| TEXAS INSTRUMENTS INCORPORATED
| Standard Linear and Logic Group
| IBIS Model of PCA9548A
| 8-CHANNEL I2C SWITCH WITH RESET
| This file contains package information for the following:
|  QFN 24-pin (RGE) package as [Component] PCA9548A_RGE
|  TSSOP 24-pin (PW) package as [Component] PCA9548A_PW
|  SOIC 24-pin (DW) package as [Component] PCA9548A_DW
|  TVSOP 24-pin (DGV) package as [Component] PCA9548A_DGV
|  SSOP 24-pin (DB) package as [Component] PCA9548A_DB
| This device can be powered at the following Vccs:
|  5 volt Vcc
|  3.3 volt Vcc
|  2.5 volt Vcc
| This file provides unique models under the [Model Selector] for each Vcc.
| For operation at a specific Vcc, select the appropriate model after each
| [Model Selector] keyword.
[IBIS Ver]   3.2
[Comment char]  |_char
[File Name]   pca9548a.ibs
[File Rev]   1.1 | a_die
[Date]   January 23, 2008
[Source]   Data created from TI-SPICE simulations at TI-SLL.
[Notes]   The following is an IBIS list for the PCA9548A.
   Please contact sllibis@ti.com with questions and
   comments concerning SLL IBIS models.
   - FILE REV HISTORY
   - 1.1 Release IBIS file on 1/23/08
   - Power clamp data has been deleted in all models except
   SDA terminator models as there is no power-clamp diode.
   - Non-monotonic data due to FET characteristics.
[Disclaimer] Property of Texas Instruments Incorporated.  Unauthorized
   reproduction and/or distribution is strictly prohibited.
   This product is protected under copyright law.
   Created  2007, (C) Copyright  2008, Texas Instruments
   Incorporated, All Rights Reserved
   UNLESS THERE IS A SIGNED, WRITTEN AGREEMENT TO THE
   CONTRARY, TEXAS INSTRUMENTS (TI) IS PROVIDING THE IBIS
   MODELS  AND WITHOUT ANY WARRANTY, EXPRESSED OR
   IMPLIED.  TI assumes no liability for:
   1) the accuracy of the IBIS models provided to your
   company;
   2) the proper functioning of these IBIS Models in your
   design or for any resulting applications; or
   3) infringement of patents, copyrights or intellectual
   property rights resulting from your use of these IBIS
   models.
   TI provides IBIS Models as a service to our customers.
   You and your company shall not distribute, sell or give
   these models to anyone else without prior written
   permission from TI.
   TI reserves the right to make changes to our products or
   to discontinue any semiconductor product or service
   without notice, and advises our customers to obtain the
   latest version of relevant information to verify, before
   placing orders, that the information being relied on is
   current.
   Please be aware that your receipt and use of the IBIS
   information provided shall serve as acceptance of these
   terms and conditions.  If you do not accept these terms,
   you should return or destroy the IBIS models and any
   other accompanying information immediately.
| Component PCA9548_RGE 24-PIN QFN
[Component]   PCA9548_RGE
[Manufacturer]   Texas Instruments, Inc.
[Package]
|   typ   min   max
R_pkg   3.700e-02   2.500e-02   5.300e-02
L_pkg   8.060e-10   5.310e-10   1.139e-09
C_pkg   1.880e-13   5.700e-14   3.100e-13
[Pin]   signal_name   model_name   R_pin   L_pin   C_pin
1   A0   PCA9548_A   3.300e-02   7.260e-10   2.460e-13
2   A1   PCA9548_A   3.200e-02   6.830e-10   2.620e-13
3   NRESET   NC   3.000e-02   6.550e-10   2.410e-13
4   SD0   PCA9548_SDX   3.000e-02   6.580e-10   2.400e-13
5   SC0   PCA9548_SCX   3.100e-02   6.770e-10   2.330e-13
6   SD1   PCA9548_SDX   3.500e-02   7.590e-10   2.490e-13
7   SC1   PCA9548_SCX   3.700e-02   7.990e-10   2.540e-13
8   SD2   PCA9548_SDX   4.500e-02   9.840e-10   2.710e-13
9   SC2   PCA9548_SCX   4.500e-02   9.870e-10   2.580e-13
10   SD3   PCA9548_SDX   4.100e-02   8.860e-10   2.340e-13
11   SC3   PCA9548_SCX   4.700e-02   1.014e-09   2.510e-13
12   GND   GND   3.600e-02   7.740e-10   2.390e-13
13   SD4   PCA9548_SDX   3.600e-02   7.870e-10   2.540e-13
14   SC4   PCA9548_SCX   3.200e-02   7.070e-10   2.350e-13
15   SD5   PCA9548_SDX   2.900e-02   6.430e-10   2.300e-13
16   SC5   PCA9548_SCX   3.000e-02   6.450e-10   2.300e-13
17   SD6   PCA9548_SDX   3.300e-02   7.100e-10   2.360e-13
18   SC6   PCA9548_SCX   3.800e-02   8.150e-10   2.570e-13
19   SD7   PCA9548_SDX   3.600e-02   7.750e-10   2.390e-13
20   SC7   PCA9548_SCX   4.700e-02   1.015e-09   2.510e-13
21   A2   PCA9548_A   4.100e-02   8.850e-10   2.360e-13
22   SCL   PCA9548_SCL   4.700e-02   1.028e-09   3.100e-13
23   SDA   PCA9548_SDA   5.300e-02   1.139e-09   2.800e-13
24   VCC   POWER   3.400e-02   7.350e-10   2.480e-13
| Component PCA9548A_PW 24-pin TSSOP
[Component]   PCA9548A_PW
[Manufacturer]   Texas Instruments, Inc.
[Package]
|   typ   min   max
R_pkg   3.900e-02   3.000e-02   4.600e-02
L_pkg   2.685e-09   2.367e-09   3.177e-09
C_pkg   3.200e-13   2.520e-13   4.340e-13
[Pin]   signal_name   model_name   R_pin   L_pin   C_pin
1   A0   PCA9548_A   3.700e-02   3.153e-09   4.340e-13
2   A1   PCA9548_A   3.400e-02   2.629e-09   3.410e-13
3   NRESET   NC   3.200e-02   2.860e-09   3.470e-13
4   SD0   PCA9548_SDX   4.200e-02   2.741e-09   2.900e-13
5   SC0   PCA9548_SCX   4.600e-02   2.600e-09   2.620e-13
6   SD1   PCA9548_SDX   4.300e-02   2.414e-09   2.660e-13
7   SC1   PCA9548_SCX   4.200e-02   2.367e-09   2.620e-13
8   SD2   PCA9548_SDX   4.400e-02   2.461e-09   2.520e-13
9   SC2   PCA9548_SCX   4.200e-02   2.543e-09   2.740e-13
10   SD3   PCA9548_SDX   3.000e-02   2.616e-09   3.320e-13
11   SC3   PCA9548_SCX   3.700e-02   2.670e-09   3.460e-13
12   GND   GND   3.900e-02   3.177e-09   4.330e-13
13   SD4   PCA9548_SDX   3.700e-02   3.111e-09   4.310e-13
14   SC4   PCA9548_SCX   3.700e-02   2.656e-09   3.450e-13
15   SD5   PCA9548_SDX   3.100e-02   2.739e-09   3.400e-13
16   SC5   PCA9548_SCX   4.200e-02   2.649e-09   2.820e-13
17   SD6   PCA9548_SDX   4.600e-02   2.532e-09   2.570e-13
18   SC6   PCA9548_SCX   4.400e-02   2.425e-09   2.660e-13
19   SD7   PCA9548_SDX   4.400e-02   2.425e-09   2.660e-13
20   SC7   PCA9548_SCX   4.600e-02   2.532e-09   2.570e-13
21   A2   PCA9548_A   4.200e-02   2.648e-09   2.820e-13
22   SCL   PCA9548_SCL   3.100e-02   2.738e-09   3.390e-13
23   SDA   PCA9548_SDA   3.600e-02   2.653e-09   3.440e-13
24   VCC   POWER   3.700e-02   3.110e-09   4.310e-13
| Component PCA9548A_DW 24-pin SOIC
[Component]   PCA9548A_DW
[Manufacturer]   Texas Instruments, Inc.
[Package]
|   typ   min   max
R_pkg   3.700e-02   3.000e-02   4.700e-02
L_pkg   5.146e-09   3.993e-09   6.885e-09
C_pkg   7.580e-13   5.120e-13   1.067e-12
[Pin]   signal_name   model_name   R_pin   L_pin   C_pin
1   A0   PCA9548_A   3.900e-02   6.885e-09   1.067e-12
2   A1   PCA9548_A   4.200e-02   5.950e-09   9.580e-13
3   NRESET   NC   4.700e-02   5.317e-09   7.910e-13
4   SD0   PCA9548_SDX   3.100e-02   4.651e-09   6.110e-13
5   SC0   PCA9548_SCX   3.000e-02   3.993e-09   5.120e-13
6   SD1   PCA9548_SDX   3.000e-02   4.083e-09   6.110e-13
7   SC1   PCA9548_SCX   3.000e-02   4.083e-09   6.110e-13
8   SD2   PCA9548_SDX   3.000e-02   3.993e-09   5.120e-13
9   SC2   PCA9548_SCX   3.100e-02   4.652e-09   6.110e-13
10   SD3   PCA9548_SDX   4.700e-02   5.317e-09   7.910e-13
11   SC3   PCA9548_SCX   4.200e-02   5.950e-09   9.590e-13
12   GND   GND   3.900e-02   6.885e-09   1.067e-12
13   SD4   PCA9548_SDX   3.900e-02   6.885e-09   1.067e-12
14   SC4   PCA9548_SCX   4.200e-02   5.950e-09   9.590e-13
15   SD5   PCA9548_SDX   4.700e-02   5.317e-09   7.910e-13
16   SC5   PCA9548_SCX   3.100e-02   4.652e-09   6.110e-13
17   SD6   PCA9548_SDX   3.000e-02   3.993e-09   5.120e-13
18   SC6   PCA9548_SCX   3.000e-02   4.083e-09   6.100e-13
19   SD7   PCA9548_SDX   3.000e-02   4.083e-09   6.100e-13
20   SC7   PCA9548_SCX   3.000e-02   3.993e-09   5.120e-13
21   A2   PCA9548_A   3.100e-02   4.651e-09   6.110e-13
22   SCL   PCA9548_SCL   4.700e-02   5.317e-09   7.910e-13
23   SDA   PCA9548_SDA   4.200e-02   5.950e-09   9.580e-13
24   VCC   POWER   3.900e-02   6.885e-09   1.067e-12
| Component PCA9548A_DGV 24-pin TVSOP
[Component]   PCA9548A_DGV
[Manufacturer]   Texas Instruments, Inc.
[Package]
|   typ   min   max
R_pkg   4.300e-02   3.900e-02   4.700e-02
L_pkg   2.601e-09   2.312e-09   3.626e-09
C_pkg   3.580e-13   2.770e-13   5.950e-13
[Pin]   signal_name   model_name   R_pin   L_pin   C_pin
1   A0   PCA9548_A   4.300e-02   3.625e-09   5.950e-13
2   A1   PCA9548_A   4.000e-02   2.656e-09   4.020e-13
3   NRESET   NC   3.900e-02   2.338e-09   3.080e-13
4   SD0   PCA9548_SDX   4.600e-02   2.354e-09   2.770e-13
5   SC0   PCA9548_SCX   4.500e-02   2.312e-09   2.850e-13
6   SD1   PCA9548_SDX   4.700e-02   2.318e-09   2.820e-13
7   SC1   PCA9548_SCX   4.700e-02   2.318e-09   2.820e-13
8   SD2   PCA9548_SDX   4.500e-02   2.312e-09   2.850e-13
9   SC2   PCA9548_SCX   4.600e-02   2.353e-09   2.780e-13
10   SD3   PCA9548_SDX   3.900e-02   2.338e-09   3.080e-13
11   SC3   PCA9548_SCX   4.100e-02   2.660e-09   4.020e-13
12   GND   GND   4.300e-02   3.625e-09   5.950e-13
13   SD4   PCA9548_SDX   4.400e-02   3.626e-09   5.940e-13
14   SC4   PCA9548_SCX   4.000e-02   2.658e-09   4.020e-13
15   SD5   PCA9548_SDX   3.900e-02   2.343e-09   3.110e-13
16   SC5   PCA9548_SCX   4.600e-02   2.353e-09   2.780e-13
17   SD6   PCA9548_SDX   4.500e-02   2.312e-09   2.850e-13
18   SC6   PCA9548_SCX   4.700e-02   2.319e-09   2.820e-13
19   SD7   PCA9548_SDX   4.700e-02   2.319e-09   2.820e-13
20   SC7   PCA9548_SCX   4.500e-02   2.312e-09   2.850e-13
21   A2   PCA9548_A   4.600e-02   2.353e-09   2.780e-13
22   SCL   PCA9548_SCL   3.900e-02   2.337e-09   3.080e-13
23   SDA   PCA9548_SDA   4.000e-02   2.658e-09   4.020e-13
24   VCC   POWER   4.400e-02   3.626e-09   5.950e-13
| Component PCA9548A_DB 24-pin SSOP
[Component]   PCA9548A_DB
[Manufacturer]   Texas Instruments, Inc.
[Package]
|   typ   min   max
R_pkg   4.500e-02   4.000e-02   4.900e-02
L_pkg   3.668e-09   3.226e-09   4.415e-09
C_pkg   4.160e-13   3.490e-13   5.070e-13
[Pin]   signal_name   model_name   R_pin   L_pin   C_pin
1   A0   PCA9548_A   4.200e-02   4.299e-09   5.030e-13
2   A1   PCA9548_A   4.000e-02   3.960e-09   4.990e-13
3   NRESET   NC   4.200e-02   3.775e-09   4.170e-13
4   SD0   PCA9548_SDX   4.700e-02   3.487e-09   3.690e-13
5   SC0   PCA9548_SCX   4.600e-02   3.347e-09   3.520e-13
6   SD1   PCA9548_SDX   4.900e-02   3.352e-09   3.710e-13
7   SC1   PCA9548_SCX   4.600e-02   3.226e-09   3.630e-13
8   SD2   PCA9548_SDX   4.700e-02   3.289e-09   3.490e-13
9   SC2   PCA9548_SCX   4.700e-02   3.347e-09   3.610e-13
10   SD3   PCA9548_SDX   4.100e-02   3.576e-09   4.090e-13
11   SC3   PCA9548_SCX   4.100e-02   3.995e-09   5.030e-13
12   GND   GND   4.500e-02   4.415e-09   5.070e-13
13   SD4   PCA9548_SDX   4.300e-02   4.337e-09   5.060e-13
14   SC4   PCA9548_SCX   4.200e-02   4.003e-09   5.040e-13
15   SD5   PCA9548_SDX   4.100e-02   3.686e-09   4.100e-13
16   SC5   PCA9548_SCX   4.800e-02   3.355e-09   3.490e-13
17   SD6   PCA9548_SDX   4.700e-02   3.301e-09   3.530e-13
18   SC6   PCA9548_SCX   4.800e-02   3.268e-09   3.660e-13
19   SD7   PCA9548_SDX   4.800e-02   3.269e-09   3.660e-13
20   SC7   PCA9548_SCX   4.700e-02   3.314e-09   3.490e-13
21   A2   PCA9548_A   4.800e-02   3.399e-09   3.550e-13
22   SCL   PCA9548_SCL   4.100e-02   3.688e-09   4.120e-13
23   SDA   PCA9548_SDA   4.200e-02   4.003e-09   5.040e-13
24   VCC   POWER   4.300e-02   4.347e-09   5.050e-13
[Series Switch Groups]
| Function Group States
On  1 /   | SDA/SCL<->SD/SC0
On  2 /   | SDA/SCL<->SD/SC1
On  3 /   | SDA/SCL<->SD/SC2
On  4 /   | SDA/SCL<->SD/SC3
On  5 /   | SDA/SCL<->SD/SC4
On  6 /   | SDA/SCL<->SD/SC5
On  7 /   | SDA/SCL<->SD/SC6
On  8 /   | SDA/SCL<->SD/SC7
[Series Pin Mapping]   pin_2   model_name   function_table_group
4   23   PCA9548_SDX_50_S   1
| 4   23   PCA9548_SDX_33_S   1
| 4   23   PCA9548_SDX_25_S   1
23   4   PCA9548_SDA_50_S   1
| 23   4   PCA9548_SDA_33_S   1
| 23   4   PCA9548_SDA_25_S   1
5   22   PCA9548_SCX_50_S   1
| 5   22   PCA9548_SCX_33_S   1
| 5   22   PCA9548_SCX_25_S   1
22   5   PCA9548_SCL_50_S   1
| 22   5   PCA9548_SCL_33_S   1
| 22   5   PCA9548_SCL_25_S   1
6   23   PCA9548_SDX_50_S   2
| 6   23   PCA9548_SDX_33_S   2
| 6   23   PCA9548_SDX_25_S   2
23   6   PCA9548_SDA_50_S   2
| 23   6   PCA9548_SDA_33_S   2
| 23   6   PCA9548_SDA_25_S   2
7   22   PCA9548_SCX_50_S   2
| 7   22   PCA9548_SCX_33_S   2
| 7   22   PCA9548_SCX_25_S   2
22   7   PCA9548_SCL_50_S   2
| 22   7   PCA9548_SCL_33_S   2
| 22   7   PCA9548_SCL_25_S   2
8   23   PCA9548_SDX_50_S   3
| 8   23   PCA9548_SDX_33_S   3
| 8   23   PCA9548_SDX_25_S   3
23   8   PCA9548_SDA_50_S   3
| 23   8   PCA9548_SDA_33_S   3
| 23   8   PCA9548_SDA_25_S   3
9   22   PCA9548_SCX_50_S   3
| 9   22   PCA9548_SCX_33_S   3
| 9   22   PCA9548_SCX_25_S   3
22   9   PCA9548_SCL_50_S   3
| 22   9   PCA9548_SCL_33_S   3
| 22   9   PCA9548_SCL_25_S   3
10   23   PCA9548_SDX_50_S   4
| 10   23   PCA9548_SDX_33_S   4
| 10   23   PCA9548_SDX_25_S   4
23   10   PCA9548_SDA_50_S   4
| 23   10   PCA9548_SDA_33_S   4
| 23   10   PCA9548_SDA_25_S   4
11   22   PCA9548_SCX_50_S   4
| 11   22   PCA9548_SCX_33_S   4
| 11   22   PCA9548_SCX_25_S   4
22   11   PCA9548_SCL_50_S   4
| 22   11   PCA9548_SCL_33_S   4
| 22   11   PCA9548_SCL_25_S   4
13   23   PCA9548_SDX_50_S   5
| 13   23   PCA9548_SDX_33_S   5
| 13   23   PCA9548_SDX_25_S   5
23   13   PCA9548_SDA_50_S   5
| 23   13   PCA9548_SDA_33_S   5
| 23   13   PCA9548_SDA_25_S   5
14   22   PCA9548_SCX_50_S   5
| 14   22   PCA9548_SCX_33_S   5
| 14   22   PCA9548_SCX_25_S   5
22   14   PCA9548_SCL_50_S   5
| 22   14   PCA9548_SCL_33_S   5
| 22   14   PCA9548_SCL_25_S   5
15   23   PCA9548_SDX_50_S   6
| 15   23   PCA9548_SDX_33_S   6
| 15   23   PCA9548_SDX_25_S   6
23   15   PCA9548_SDA_50_S   6
| 23   15   PCA9548_SDA_33_S   6
| 23   15   PCA9548_SDA_25_S   6
16   22   PCA9548_SCX_50_S   6
| 16   22   PCA9548_SCX_33_S   6
| 16   22   PCA9548_SCX_25_S   6
22   16   PCA9548_SCL_50_S   6
| 22   16   PCA9548_SCL_33_S   6
| 22   16   PCA9548_SCL_25_S   6
17   23   PCA9548_SDX_50_S   7
| 17   23   PCA9548_SDX_33_S   7
| 17   23   PCA9548_SDX_25_S   7
23   17   PCA9548_SDA_50_S   7
| 23   17   PCA9548_SDA_33_S   7
| 23   17   PCA9548_SDA_25_S   7
18   22   PCA9548_SCX_50_S   7
| 18   22   PCA9548_SCX_33_S   7
| 18   22   PCA9548_SCX_25_S   7
22   18   PCA9548_SCL_50_S   7
| 22   18   PCA9548_SCL_33_S   7
| 22   18   PCA9548_SCL_25_S   7
19   23   PCA9548_SDX_50_S   8
| 19   23   PCA9548_SDX_33_S   8
| 19   23   PCA9548_SDX_25_S   8
23   19   PCA9548_SDA_50_S   8
| 23   19   PCA9548_SDA_33_S   8
| 23   19   PCA9548_SDA_25_S   8
20   22   PCA9548_SCX_50_S   8
| 20   22   PCA9548_SCX_33_S   8
| 20   22   PCA9548_SCX_25_S   8
22   20   PCA9548_SCL_50_S   8
| 22   20   PCA9548_SCL_33_S   8
| 22   20   PCA9548_SCL_25_S   8
| Model PCA9548_A
[Model Selector]   PCA9548_A
PCA9548_A_50   5 volt Vcc
PCA9548_A_33   3.3 volt Vcc
PCA9548_A_25   2.5 volt Vcc
| Model PCA9548_SDX
[Model Selector]   PCA9548_SDX
PCA9548_SDX_50   5 volt Vcc
PCA9548_SDX_33   3.3 volt Vcc
PCA9548_SDX_25   2.5 volt Vcc
| Model PCA9548_SDX_S
[Model Selector]   PCA9548_SDX_S
PCA9548_SDX_50_S   5 volt Vcc
PCA9548_SDX_33_S   3.3 volt Vcc
PCA9548_SDX_25_S   2.5 volt Vcc
| Model PCA9548_SCL
[Model Selector]   PCA9548_SCL
PCA9548_SCL_50   5 volt Vcc
PCA9548_SCL_33   3.3 volt Vcc
PCA9548_SCL_25   2.5 volt Vcc
| Model PCA9548_SCL_S
[Model Selector]   PCA9548_SCL_S
PCA9548_SCL_50_S   5 volt Vcc
PCA9548_SCL_33_S   3.3 volt Vcc
PCA9548_SCL_25_S   2.5 volt Vcc
| Model PCA9548_SDA
[Model Selector]   PCA9548_SDA
PCA9548_SDA_50   5 volt Vcc
PCA9548_SDA_33   3.3 volt Vcc
PCA9548_SDA_25   2.5 volt Vcc
| Model PCA9548_SDA_S
[Model Selector]   PCA9548_SDA_S
PCA9548_SDA_50_S   5 volt Vcc
PCA9548_SDA_33_S   3.3 volt Vcc
PCA9548_SDA_25_S   2.5 volt Vcc
| Model PCA9548_SCX
[Model Selector]   PCA9548_SCX
PCA9548_SCX_50   5 volt Vcc
PCA9548_SCX_33   3.3 volt Vcc
PCA9548_SCX_25   2.5 volt Vcc
| Model PCA9548_SCX_S
[Model Selector]   PCA9548_SCX_S
PCA9548_SCX_50_S   5 volt Vcc
PCA9548_SCX_33_S   3.3 volt Vcc
PCA9548_SCX_25_S   2.5 volt Vcc
[Model]   PCA9548_SDX_50_S
Model_type  Series_switch
| variable   typ   min   max
C_comp   0   0   0
[Temperature Range]   40   100   -40
| Ambient temperature   25   85   -40
[Voltage range]   5   4.5   5.5
[On]
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[Off]
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[Model]   PCA9548_SDX_33_S
Model_type  Series_switch
| variable   typ   min   max
C_comp   0   0   0
[Temperature Range]   40   100   -40
| Ambient temperature   25   85   -40
[Voltage range]   3.3   3   3.6
[On]
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[Off]
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[Model]   PCA9548_SDX_25_S
Model_type  Series_switch
| variable   typ   min   max
C_comp   0   0   0
[Temperature Range]   40   100   -40
| Ambient temperature   25   85   -40
[Voltage range]   2.5   2.3   2.7
[On]
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[Off]
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[Model]   PCA9548_SCL_50_S
Model_type  Series_switch
| variable   typ   min   max
C_comp   0   0   0
[Temperature Range]   40   100   -40
| Ambient temperature   25   85   -40
[Voltage range]   5   4.5   5.5
[On]
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[Off]
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[Model]   PCA9548_SCL_33_S
Model_type  Series_switch
| variable   typ   min   max
C_comp   0   0   0
[Temperature Range]   40   100   -40
| Ambient temperature   25   85   -40
[Voltage range]   3.3   3   3.6
[On]
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[Off]
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[Model]   PCA9548_SCL_25_S
Model_type  Series_switch
| variable   typ   min   max
C_comp   0   0   0
[Temperature Range]   40   100   -40
| Ambient temperature   25   85   -40
[Voltage range]   2.5   2.3   2.7
[On]
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[Off]
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[Model]   PCA9548_SDA_50_S
Model_type  Series_switch
| variable   typ   min   max
C_comp   0   0   0
[Temperature Range]   40   100   -40
| Ambient temperature   25   85   -40
[Voltage range]   5   4.5   5.5
[On]
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[Off]
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[Model]   PCA9548_SDA_33_S
Model_type  Series_switch
| variable   typ   min   max
C_comp   0   0   0
[Temperature Range]   40   100   -40
| Ambient temperature   25   85   -40
[Voltage range]   3.3   3   3.6
[On]
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[Off]
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[Model]   PCA9548_SDA_25_S
Model_type  Series_switch
| variable   typ   min   max
C_comp   0   0   0
[Temperature Range]   40   100   -40
| Ambient temperature   25   85   -40
[Voltage range]   2.5   2.3   2.7
[On]
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[Off]
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[Model]   PCA9548_SCX_50_S
Model_type  Series_switch
| variable   typ   min   max
C_comp   0   0   0
[Temperature Range]   40   100   -40
| Ambient temperature   25   85   -40
[Voltage range]   5   4.5   5.5
[On]
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[Off]
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[Model]   PCA9548_SCX_33_S
Model_type  Series_switch
| variable   typ   min   max
C_comp   0   0   0
[Temperature Range]   40   100   -40
| Ambient temperature   25   85   -40
[Voltage range]   3.3   3   3.6
[On]
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[Off]
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[Model]   PCA9548_SCX_25_S
Model_type  Series_switch
| variable   typ   min   max
C_comp   0   0   0
[Temperature Range]   40   100   -40
| Ambient temperature   25   85   -40
[Voltage range]   2.5   2.3   2.7
[On]
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[Off]
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| Models and submodels in the file (27): PCA9548_A_50 (Input), PCA9548_A_33 (Input), PCA9548_A_25 (Input), PCA9548_SDX_50_S (Series_switch), PCA9548_SDX_50 (Terminator), PCA9548_SDX_33_S (Series_switch), PCA9548_SDX_33 (Terminator), PCA9548_SDX_25_S (Series_switch), PCA9548_SDX_25 (Terminator), PCA9548_SCL_50_S (Series_switch), PCA9548_SCL_50 (Terminator), PCA9548_SCL_33_S (Series_switch), PCA9548_SCL_33 (Terminator), PCA9548_SCL_25_S (Series_switch), PCA9548_SCL_25 (Terminator), PCA9548_SDA_50_S (Series_switch), PCA9548_SDA_50 (Terminator), PCA9548_SDA_33_S (Series_switch), PCA9548_SDA_33 (Terminator), PCA9548_SDA_25_S (Series_switch), PCA9548_SDA_25 (Terminator), PCA9548_SCX_50_S (Series_switch), PCA9548_SCX_50 (Terminator), PCA9548_SCX_33_S (Series_switch), PCA9548_SCX_33 (Terminator), PCA9548_SCX_25_S (Series_switch), PCA9548_SCX_25 (Terminator)
